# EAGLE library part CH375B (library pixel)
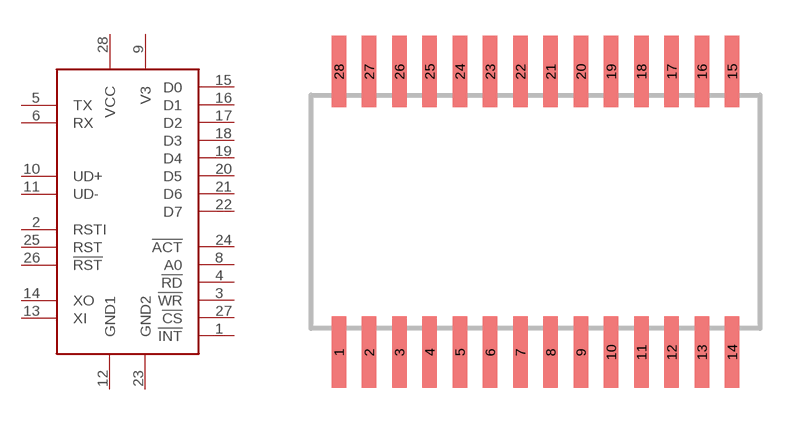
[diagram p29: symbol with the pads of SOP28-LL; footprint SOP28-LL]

Designator prefix -

## CH375B  [SOP28-LL]
1  !INT
2  RSTI
3  !WR
4  !RD
5  TX
6  RX
8  A0
9  V3
10  UD+
11  UD-
12  GND1
13  XI
14  XO
15  D0
16  D1
17  D2
18  D3
19  D4
20  D5
21  D6
22  D7
23  GND2
24  !ACT
25  RST
26  !RST
27  !CS
28  VCC

## Footprint SOP28-LL (pad centres in mm)
SMALL OUTLINE PACKAGE
smd 0.6 x 3: 1 -8.255,-5.9; 2 -6.985,-5.9; 3 -5.715,-5.9; 4 -4.445,-5.9; 5 -3.175,-5.9; 6 -1.905,-5.9; 7 -0.635,-5.9; 8 0.635,-5.9; 9 1.905,-5.9; 10 3.175,-5.9; 11 4.445,-5.9; 12 5.715,-5.9; 13 6.985,-5.9; 14 8.255,-5.9; 15 8.255,5.9; 16 6.985,5.9; 17 5.715,5.9; 18 4.445,5.9; 19 3.175,5.9; 20 1.905,5.9; 21 0.635,5.9; 22 -0.635,5.9; 23 -1.905,5.9; 24 -3.175,5.9; 25 -4.445,5.9; 26 -5.715,5.9; 27 -6.985,5.9; 28 -8.255,5.9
